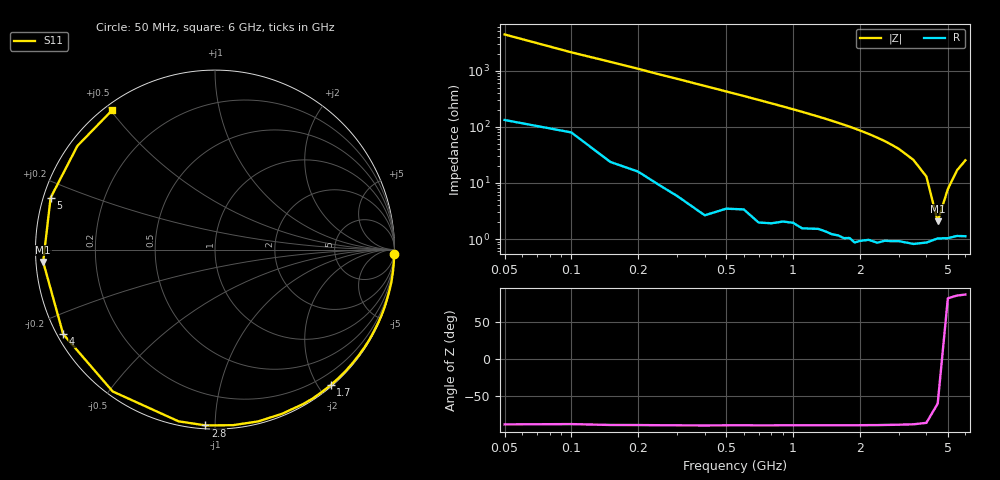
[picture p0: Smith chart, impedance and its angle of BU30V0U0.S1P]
! Infineon Technologies  Discrete & RF Semiconductors
! BB 833
! Si Tuning Diode in SOD323
! VR = 30 V
! S-Parameters:  June  1999
# GHz  S  MA  R  50
!  f  S11
! GHz  MAG  ANG
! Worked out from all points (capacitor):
!   34 points, 50 MHz to 6 GHz, reference 50 ohm
!   read as one part to ground: C = 740 fF near 50 MHz
!   lowest |Z| = 2.06 ohm at 4.5 GHz (marker M1)
!   series resonance near 4.594 GHz, so ESL is about 1.6 nH
!   S11 on the Smith chart (normalised r, x): 50 MHz: 3, -88; 1.7 GHz: 0.02, -2.17; 2.8 GHz: 0.02, -0.95; 4 GHz: 0.02, -0.26; 5 GHz: 0.02, +0.15; 6 GHz: 0.02, +0.50
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0.05  0.9993 -1.3
0.25  0.9988 -6.7
0.4  0.9991 -10.7
0.6  0.9974 -16.1
0.7  0.9979 -18.9
0.8  0.9973 -21.7
1  0.9956 -27.4
1.1  0.9958 -30.3
1.2  0.995 -33.4
1.3  0.9941 -36.4
1.4  0.9938 -39.5
1.5  0.9935 -42.8
1.6  0.9929 -46.1
1.7  0.9928 -49.5
1.8  0.9917 -52.9
1.9  0.9923 -56.5
2  0.9907 -60.2
2.2  0.988 -67.8
2.4  0.9871 -75.9
2.6  0.9834 -84.2
2.8  0.9809 -93.1
3  0.9781 -102.0
3.5  0.9744 -125.8
4  0.9681 -150.9
4.5  0.9599 -175.9
5  0.9603 162.5
5.5  0.96 143.0
6  0.9649 126.5
